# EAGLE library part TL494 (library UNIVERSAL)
TL494N upraveny pre priepustny menic. DIL16
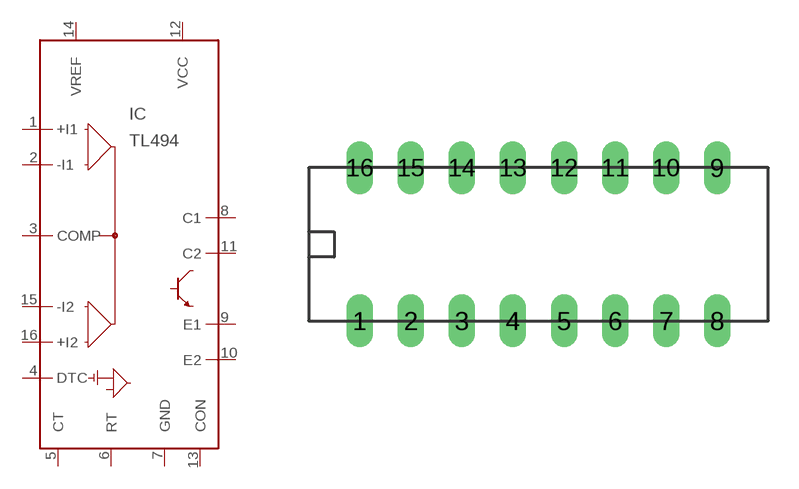
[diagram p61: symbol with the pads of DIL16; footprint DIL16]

Designator prefix IC

## TL494  [DIL16]
1  +I1  in
2  -I1  in
3  COMP  pas
4  DTC  in
5  CT  in
6  RT  in
7  GND  pwr
8  C1  pas
9  E1  pas
10  E2  pas
11  C2  pas
12  VCC  pwr
13  CON  out
14  VREF  in
15  -I2  in
16  +I2  in

## Footprint DIL16 (pad centres in mm)
drill 0.813 pad 1.27 long: 1 0,1.27; 2 2.54,1.27; 3 5.08,1.27; 4 7.62,1.27; 5 10.16,1.27; 6 12.7,1.27; 7 15.24,1.27; 8 17.78,1.27; 9 17.78,8.89; 10 15.24,8.89; 11 12.7,8.89; 12 10.16,8.89; 13 7.62,8.89; 14 5.08,8.89; 15 2.54,8.89; 16 0,8.89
